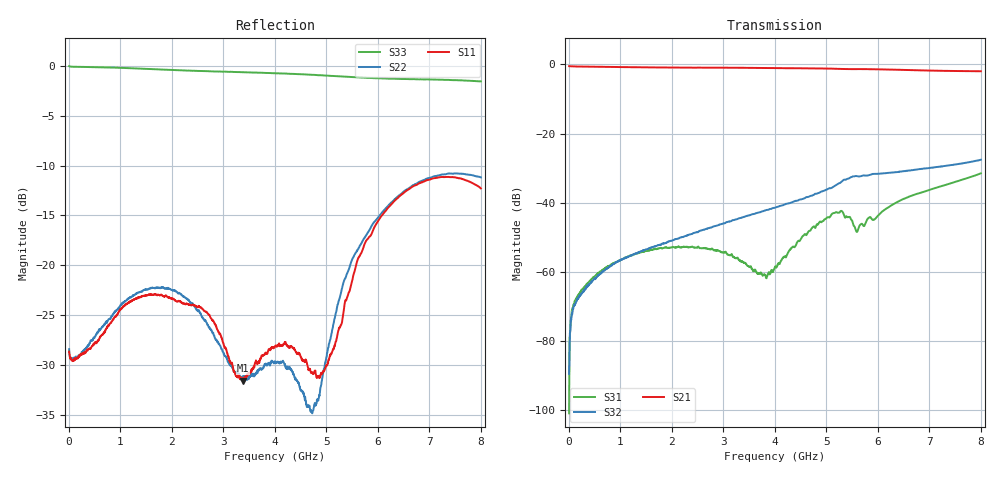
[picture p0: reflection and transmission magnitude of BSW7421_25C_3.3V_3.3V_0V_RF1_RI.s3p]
! Product: BSW7421
! Temp: 25C
! VDD: 3.300
! Control_Hi: 3.300
! Control_Lo: 0.000
! Logic State: RF1
! Port 1: RFC
! Port 2: RF1
! Port 3: RF2
! V1 = 3.30
! V2 = 0.00
! V3 = 0.00
! V4 = 0.00
# Hz S  RI  R 50
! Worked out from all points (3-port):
!   1601 points, 5 MHz to 8.005 GHz, reference 50 ohm
!   strongest paths, dB at 5 MHz, 2.005 GHz, 4.005 GHz, 6.005 GHz, 8.005 GHz:
!     S21: -0.5, -0.9, -1.1, -1.4, -2.0
!     S32: -89.5, -51.0, -41.4, -31.6, -27.6
!     S31: -100.9, -52.9, -58.6, -43.7, -31.5
!   lowest |S11| = -31.6 dB at 3.38 GHz (marker M1), VSWR 1.05, Z = 52.1 + j1.7 ohm
!   |S11| at or under -10 dB: start of sweep to end of sweep
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5000000  0.0365 -0.005  0.9413 -0.0135  3.03e-05 5.17e-05
         0.9415 -0.0133  0.0376 -0.00501  1.46e-05 3.29e-05
         -8.45e-06 -3.24e-06  -4.01e-06 3.34e-05  0.9997 -0.0103
8.95e8  -0.0394 -0.0383  0.0962 -0.9117  0.00135 -0.000231
        0.0962 -0.9116  -0.0372 -0.0454  0.00131 0.000264
        0.00135 -0.000222  0.00131 0.000258  0.0252 -0.9824
1.8e9  -0.034 0.0624  -0.8786 -0.1939  -8.55e-05 -0.00219
       -0.8786 -0.1938  -0.0555 0.0543  0.00175 -0.00184
       -7.61e-05 -0.00219  0.00175 -0.00182  -0.9601 -0.0599
2.635e9  0.0347 0.0476  -0.3876 0.8093  -0.00217 -0.000541
         -0.3874 0.8093  0.0244 0.0467  -0.000773 -0.00401
         -0.00213 -0.000543  -0.000778 -0.00402  -0.2561 0.9091
3.38e9  0.0206 0.0163  0.6168 0.644  -0.00104 0.000931
        0.6167 0.6439  0.0195 0.0191  -0.0055 -0.00278
        -0.00102 0.000954  -0.0055 -0.00279  0.7366 0.573
4.005e9  0.0362 0.0152  0.865 -0.1781  -0.00113 0.000337
         0.8654 -0.1783  0.0277 0.017  -0.00806 0.00269
         -0.00113 0.000349  -0.00805 0.00267  0.8643 -0.32
4.84e9  -0.00407 -0.0274  0.0134 -0.873  -0.00198 0.00444
        0.0134 -0.8729  -0.0111 -0.018  -0.00238 0.0136
        -0.00198 0.00444  -0.00237 0.0136  -0.1964 -0.879
5.795e9  -0.0315 0.1309  -0.8523 -0.0355  0.00483 0.00304
         -0.8523 -0.0349  -0.0194 0.1426  0.0245 0.00322
         0.00485 0.00303  0.0245 0.00323  -0.7946 0.3616
6.825e9  0.2593 -0.00322  0.0488 0.8176  0.00792 -0.0113
         0.0493 0.8179  0.2633 0.0128  0.00189 -0.0307
         0.00789 -0.0114  0.0019 -0.0305  0.5682 0.6436
8.005e9  -0.1072 -0.2183  0.7365 -0.2994  -0.0261 -0.00532
         0.736 -0.2998  -0.0344 -0.2742  -0.0418 0.00299
         -0.0261 -0.00523  -0.0417 0.00306  0.4216 -0.7247
